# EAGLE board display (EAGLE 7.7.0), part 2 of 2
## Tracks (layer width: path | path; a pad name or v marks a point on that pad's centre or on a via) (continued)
N$131 (continued)
  Top 0.2: 54.6,23.5 1.9,23.5 1.9,23.4 | 1.9,23.4 2.3,23.3 | 2.3,23.3 2.2,23.1 | 2.2,23.1 2.2,23.2 | 2.2,23.2 1.9,23.4 | 2.3,23.3 2.3,23 2.2,22.8 | 1.9,23.4 1.9,20 3.3,20 3.3,22.9 | 2.7,22.1 2.7,22.3 3.3,22.9 | 3.6,23.3 3.7,23.3 3.3,22.9 | 3.6,23.3 3,22.7 2.4,22.7 2.2,22.9 | 2.2,22.9 1.9,23.2 1.9,21.6 | 1.9,21.6 1.9,20.8 2,20.7 2.2,20.7 2.6,20.3 2.6,20.7 | 2.6,22.1 2.6,22.6 3.1,23.1 | 3.1,23.1 3.1,23 | 3.1,23 3.1,22.3 | 3.1,22.3 3,22.2 3,22 2.9,22 2.8,22.1 2.8,23.1 2.9,23.2 | 2.6,21.6 1.9,21.6 | 1.9,21.6 2.3,21.8 2.2,23.2 | 2.2,23.2 2.1,23.2 | 2.1,23.2 1.9,23.4 | 1.9,23.4 54,23.4 | 54,23.4 56.3,23.4 | 56.3,23.4 56.3,26.2 54.4,26.2 54.4,23.5 54.5,23.5 54.6,23.6 | 54.6,25.7 54.6,25.9 54.5,26 56.2,26 56.2,25.6 | 56.2,24.4 56.2,24.2 | 56.2,24.2 56.2,23.5 | 56.2,23.5 54.7,23.5 54.6,23.6 | 54.6,23.6 54.6,23.9 | 54.6,23.9 54.6,24 | 54.6,24.1 54.6,24.4 | 54.6,24.4 54.6,25.7 | 54.6,25.7 54.8,25.9 55.9,25.9 56,25.8 56,24.1 | 56,24.1 56,23.7 54.7,23.7 54.7,23.8 54.6,23.9 | 54.6,23.9 56.1,23.9 56.1,24.1 56.2,24.2 | 56.2,24.2 56.1,24.2 | 56.1,24.2 55.6,24.2 | 55.6,24.2 54.7,24.2 54.6,24.1 | 56,24.1 54.7,24.1 54.6,24 | 54.6,24 54.6,24.1 | 54.6,24.4 54.8,24.4 | 54.8,24.4 56.2,24.4 | 56.2,24.4 56.2,25.6 | 56.2,25.6 56.1,25.7 55.9,25.7 | 55.9,25.7 55.5,25.7 | 55.5,25.7 54.8,25.7 | 54.8,25.7 54.7,25.6 55,25.6 | 55,25.6 55.2,25.6 | 55.2,25.6 55.3,25.6 | 55.3,25.6 55.8,25.6 | 55.8,25.6 55.9,25.7 | 55.9,25.7 56.1,25.9 56.1,25.5 | 56.1,24.2 56.1,25.5 | 56.1,25.5 55.9,25.7 | 55.9,25.7 55.9,25.5 | 55.9,24 55.9,25.5 | 55.9,25.5 55.8,25.6 | 55.8,25.6 55.8,25.4 | 55.8,23.8 55.8,25.4 | 55.8,25.4 55.5,25.7 | 55.5,25.7 55.5,24.3 55.6,24.2 | 55.6,24.2 55.6,25.7 55.5,25.8 55.3,25.6 | 55.3,25.6 55.3,24.4 55.4,24.3 55.4,25.4 55.2,25.6
  Top 0.2: 55.2,25.6 55.2,24.4 55.3,24.3 55.3,25.3 55,25.6 | 55,25.6 55,25.5 | 55,24.3 55,25.5 | 55,25.5 54.8,25.7 | 54.8,25.7 54.8,24.4 | 56.3,23.4 56.3,23.3 | R7A.2 2.4,22.95 2.65,23.2 2.9,23.2 | 2.9,23.2 34.4,23.2 | 34.4,23.2 34.5,23.2 | 34.5,23.2 34.6,23.3 54.3,23.3 | 54.3,23.3 54.4,23.3 | 55.5,23.3 56.3,23.3 | 54.35,23.45 54.4,23.3 | 54.4,23.3 55.5,23.3 | 55.5,23.3 55.5,24.62 JP16.7 54.3,23.42 54.3,23.3 | 2.4,21.9 2.1,23.2 | 2.1,23.2 2.2,23.3 | 2.2,23.3 3.1,23.3 3.1,23.1 | 3.1,20.3 3.1,20.1 2.6,20.7 | 2.6,20.7 2.6,22.1 | 2.6,22.1 2.2,23.3 | 2.9,23.2 2.9,22.8 | 2.9,22.1 2.9,22.8 | 2.9,22.8 2.6,23.1 2.2,23.1 | 2.2,23.1 2,22.9 2,22.1 2.2,22.1 2.2,22.9 | 2.2,22.9 2.6,22.9 2.7,22.8 | 34.2,23.3 34.3,23.3 34.4,23.2 | 34.5,23.2 56.3,23.2 56.3,23.3 | 56.3,23.4 56.2,23.5 | 54.6,24 54,23.4 | 3.6,23.3 3.4,23.3 3.1,23 | 3.1,22.3 3.1,20.3 | 3.1,20.3 2.9,20.1 2.1,20.1 2,20.2
N$134  (1 unrouted)
  Top 0.2: 58.2,26.8 58.4,26.6 | 58.4,26.6 58.6,26.4 | 56.9,26.9 57.1,26.7 | 57.7,26.1 57.1,26.7 | 57.1,26.7 57.3,26.7 57.3,23.2 58.5,23.2 58.6,23.3 | 58.6,23.3 58.7,23.4 58.7,26.5 58.3,26.9 57.5,26.9 57.5,26.8 | 57.5,26.8 57.5,23.4 57.6,23.3 58.3,23.3 | 58.3,23.3 58.6,23.3 | 58.6,23.3 58.6,26.3 58.2,26.7 58.1,26.7 | 58.1,26.7 57.8,26.7 | 57.8,26.7 57.7,26.7 57.7,23.4 57.9,23.4 | 58,23.4 58,23.2 | 58,23.2 58.8,23.2 58.8,26.6 58.4,27 1.1,27 1.1,19.4 | 1.1,19.4 1.1,16.7 3.2,16.7 3.2,18.8 1.4,18.8 1.3,18.9 | R6B.2 1.45,17.8 1.2,18.05 1.2,19 | 1.2,19 1.2,23.55 | 57.65,25.2 57.9,24.95 | 1.3,18.9 1.2,19 | 1.3,18.9 1.3,17 1.1,16.8 | 1.1,16.8 1.1,18 | 1.5,16.8 1.1,16.8 | 58,26.7 58,26.6 | 58,26.6 58,24.82 JP16.6 | 58,23.2 57.4,23.2 57.4,26.8 1.5,26.8 | 1.5,26.8 1.2,26.8 | 1.1,26.9 1.2,26.8 | 1.2,26.8 1.2,26.5 | 1.2,26.5 1.5,26.8 | 1.2,26.5 1.2,18.9 1.4,18.7 | 57.9,23.4 58,23.4 | 58,23.4 58,26.3 57.5,26.8 | 57.5,26.8 57.7,26.8 57.8,26.7 | 57.8,26.7 57.8,23.5 57.9,23.4 | 58,23.4 58.1,23.4 | 58.1,23.4 58.2,23.4 | 58.2,23.4 58.3,23.3 | 58.3,23.3 58.3,26.5 58.2,26.6 58.2,23.5 58.1,23.4 | 58.2,23.4 58.4,23.4 58.4,26.2 | 58.4,26.2 58.5,26.3 | 1.1,19.4 1.8,18.7 1.7,18.7 1.3,19.1 | 58.1,26.7 58,26.6 | 58.4,26.6 58.4,26.2
N$135
  Top 0.2: 2,24.8 2,24.2 | 2,24.2 1.9,24.2 1.9,26.1 53.7,26.1 53.7,24.2 2,24.2
N$137
  Top 0.2: 8.1,19.1 13.1,19.1 | 13.7,19.1 13.1,19.1 | 13.1,19.1 12.8,19.4 12.6,19.4 12.4,19.2
N$138
  Top 0.2: 8.1,18.9 13.7,18.9
N$139
  Top 0.2: 8.1,18.8 13.5,18.8
N$140
  Top 0.2: 8.1,18.4 13.1,18.4 13.3,18.6 8.5,18.6 8.4,18.5 8.4,18.4 8.3,18.3 | 13,18.3 8.3,18.3 | 8.3,18.3 8.1,18.1 12.8,18.1 | 12.8,18.1 12.9,18.2 | 12.8,18.1 12.7,18 8.4,18 8.3,17.9
N$141
  Top 0.2: 13.8,17.7 14.5,17.7 | 15.6,17.7 14.5,17.7 | 14.5,17.7 14.3,17.9
N$142
  Top 0.2: 39.2,19.1 43.4,19.1 44,19.7 | 44,19.7 43.3,19.7 | 43.3,19.7 43.2,19.7 42.7,19.2 42.8,19.2 43.3,19.7 | 44,19.7 44.1,19.7 43.6,19.2 | 43.6,19.2 43,19.2 43.4,19.6 43.6,19.6 | 43.7,19.6 43.6,19.6 | 43.6,19.6 43.3,19.3 43.5,19.3 43.6,19.2 | 43.6,19.2 43.7,19.2 | 43.7,19.2 43.8,19.3 43.8,19.1 38.8,19.1 38.7,19 | 43.7,19.2 43.7,19 43.8,18.9 38.9,18.9 38.8,18.8 38.7,18.8
N$143
  Top 0.2: 24.5,17.7 26,17.7
N$144
  Top 0.2: 62.1,22.4 66.6,22.4 66.8,22.2 62,22.2 62,22.3 61.9,22.3 61.8,22.2
N$145
  Top 0.2: 46.5,17.5 46.1,17.5
N$146
  Top 0.2: 49.9,17.5 54.7,17.5 55.2,18
N$147
  Top 0.2: 66,9 65.7,9 65.6,8.9 65.6,6.6 64.9,5.9 63.5,5.9 63.4,5.8 63.4,4.6 63.1,4.3 60.9,4.3 60.8,4.2 60.8,0.3 73.6,0.3 | 73.7,8.8 73.7,8.5 73.7,0.3 73.6,0.3 | 73.6,0.3 73.6,8.7 73.7,8.8 | 73.7,8.8 65.8,8.8 | 65.7,8.8 65.8,8.8 | 65.8,8.8 66,9 | 66,9 73.6,9 73.7,8.9 73.7,8.8
N$148
  Top 0.2: 60.8,19.3 66.9,19.3 67.7,18.5 60.5,18.5 | 60.5,18.5 60.3,18.7 60.5,18.7 | 59.6,17.4 60.6,17.4 60.8,17.6 67.3,17.6 67.4,17.5 | 67.4,17.5 67.5,17.5 67.6,17.4 67.5,17.4 | 67.5,17.4 67.4,17.5 | 67.5,17.4 67.6,17.3 67.6,16.8 | 67.6,16.8 67.9,16.8 | 69.2,16.8 69.2,17.2 69,17.4 69,18.9 | 69,18.9 68.6,18.9 | 68.6,18.9 67.5,18.9 67,19.4 60.8,19.4 60.3,18.9 | 60.3,18.9 60,18.6 | 67.6,18.7 67.3,18.7 | 67.3,18.7 60.5,18.7 | 60.5,18.7 60.3,18.9 | 60.3,18.9 60.5,18.9 | 60.5,18.9 67.1,18.9 67.3,18.7 | 67.3,18.7 67.3,18.8 67,19.1 60.7,19.1 60.5,18.9 | 60.5,18.9 60.5,19 60.7,19.2 | 60.5,18.5 60.1,18.5 | 67.7,17.3 67.7,16.9 67.6,16.8 | 67.6,16.8 67.6,16.5 69.2,16.5 69.2,16.8 | 69.2,16.8 67.9,16.8 | 67.9,16.8 67.8,16.7 | 67.8,16.7 68.8,16.7 | 68.8,16.7 68.9,16.6 69,16.6 69.1,16.7 68.8,16.7 | 67.8,16.7 67.7,16.6 | 68.6,18.8 68.6,18.9 | 69,18.9 69.1,18.9 69.1,17.2
N$149
  Top 0.2: 60,18.4 67.2,18.4 67.7,17.9 60,17.9 59.9,18 59.9,18.2 60,18.3 67.1,18.3 67.4,18 60.1,18 60,18.1 67.1,18.1
N$150
  Top 0.2: 59.9,17.9 59.9,17.6 | 59.9,17.6 59.8,17.5 | 59.9,17.6 60.7,17.6 60.9,17.8 | 60.9,17.8 67.5,17.8 67.7,17.6 67.4,17.6 67.3,17.7 | 60.9,17.8 60,17.8
N$151
  Top 0.2: 71.1,21.5 71,21.5 70.5,22 70.5,23.2 | 70.5,23.2 70.1,23.6 70.1,26.2 70.5,26.2 | 70.5,26.2 70.7,26.2 | 70.7,26.2 70.8,26.2 | 70.8,26.2 71.8,26.2 71.9,26.1 71.9,20.2 71.9,20.1 | 71.9,20.1 70.5,20.1 | 70.5,20.1 70.5,22.1 70.6,22.2 | 70.8,26.2 70.8,23.3 | 70.8,23.3 70.8,22 | 70.7,26.2 70.7,21.9 | 70.5,26.2 70.5,23.5 | 70.5,23.5 70.5,23.2 | 70.5,23.2 70.6,23.1 | 70.3,26.1 70.3,23.7 70.5,23.5 | 70.8,23.3 70.6,23.3 70.2,23.7 | 70.7,20.5 70.7,20.3 70.5,20.1 | 70.5,20.1 70.6,20 71.9,20 71.9,20.1
N$152
  Top 0.2: 71.7,26.1 71.7,20.7 71.6,20.6
N$153
  Top 0.2: 71.5,26.1 71.5,20.6
N$154
  Top 0.2: 71.4,26.1 71.4,21
N$155
  Top 0.2: 71.2,26.1 71.2,21.8 71.1,21.7
N$156
  Top 0.2: 71,26.1 71,21.8
N$157
  Top 0.2: 63.9,4.8 63.8,4.8 63,4 63.2,4 63.6,4.4
N$158
  Top 0.2: 66.8,20.5 67.6,20.5 67.7,20.4
N$159
  Top 0.2: 67.8,20.7 66.8,20.7
N$160
  Top 0.2: 67.8,20.9 66.3,20.9
N$161
  Top 0.2: 66.8,21.1 67.7,21.1 67.8,21
N$162
  Top 0.2: 67.8,21.3 66.7,21.3
N$163
  Top 0.2: 66.7,21.5 67.7,21.5
N$164
  Top 0.2: 67.9,21.7 66.8,21.7
N$166
  Top 0.2: 65.8,6.5 65,5.7 65.1,5.7 65.6,6.2 65.6,6 65.4,5.8 65.7,5.8 65.8,5.9
N$167
  Top 0.2: 40.2,20.9 39.9,20.9
N$168  (1 unrouted)
  Top 0.2: 4.7,20.5 4.7,20.1 5.6,20.1 5.7,20 | 4.8,21.4 4.8,21.7 4.5,22 4.5,22.4 4.6,22.4 | R7A.1 5.2,21.18 LED6.10 8.2,21.18 8.2,22.5 | 13.3,22.5 13.8,22.5 | 13.8,22.5 16.5,22.5 | 16.5,22.5 16.6,22.5 | 16.7,22.5 18.4,22.5 | 18.4,22.5 18.4,21.2 | 18.4,21.2 17.69,21.2 LED5.10 18.4,21.18 18.4,21.2 | 18.8,22.5 18.9,22.5 | 18.9,22.5 26.7,22.5 | 26.7,22.5 28.6,22.5 | 28.6,22.5 28.6,22.2 | LED4.10 28.6,21.18 28.6,22.2 | 28.6,22.5 28.9,22.5 | 29.1,22.5 36.9,22.5 | 36.9,22.5 38.8,22.5 | 38.8,22.5 38.8,21.2 | 38.8,21.2 38.09,21.2 LED3.10 38.8,21.18 38.8,21.2 | 39.4,22.5 47,22.5 | 47.2,22.5 49,22.5 | 49,22.5 49,21.2 | 49,21.2 48.29,21.2 LED2.10 49,21.18 49,21.2 | 49,22.5 49.3,22.5 | 58.9,22.5 59.2,22.5 | 59.2,22.1 59.2,21.4 | 59.2,21.2 58.49,21.2 LED1.10 | 4.7,22.4 8.1,22.4 8.2,22.5 | 8.2,22.5 4.5,22.5 | 4.5,22.5 4.5,20 5.7,20 | 5.7,20 5.8,20 | 5.8,20 6.2,20.4 12.4,20.4 13.1,21.1 13.1,21.8 13.8,22.5 | 4.7,22.4 4.7,22.2 8.1,22.2 8.1,22 4.8,22 4.7,22.1 4.7,22.3 4.6,22.4 | 8.2,22.5 13.3,22.5 | 13.3,22.5 13.5,22.3 13.4,22.3 13.3,22.4 | 4.7,22.4 4.6,22.4 | 4.6,22.4 4.5,22.5 | 4.5,22.5 4.5,22.6 | 59.2,22.5 60.4,22.5 59.2,21.2 | 59.2,22.5 59.2,22.1 | 59.2,22.1 59.1,22 58.4,22 58,21.6 57.1,22.5 58.9,22.5 | 58.9,22.5 59.1,22.3 57.5,22.3 57.4,22.4 57.4,22.3 57.7,22 59,22 59.1,22.1 57.7,22.1 57.7,22.2 | 48.8,21.8 49.5,22.5 | 49.5,22.5 49.3,22.5 | 49.3,22.5 49.1,22.3 48.3,22.3 47.7,21.7 47.7,21.8 47,22.5 | 47,22.5 47.2,22.5 | 47.2,22.5 47.7,22 48.7,22 48.9,22.2 48.9,22.1 48.8,22 47.9,22 47.5,22.4 48.7,22.4 48.7,22.1 47.9,22.1 47.7,22.3 48.5,22.3 48.6,22.2 | 38.4,21.8 38.7,21.8 39.4,22.5 | 39.4,22.5 38.8,22.5 | 36.9,22.5 37.6,21.8 37.6,21.9 37.5,22 38.7,22 39.1,22.4 37.3,22.4 37.3,22.3 37.4,22.2
  Top 0.2: 37.4,22.2 37.5,22.1 37.4,22.1 37.1,22.4 38.5,22.4 38.7,22.2 37.4,22.2 | 27.6,21.7 27.5,21.7 26.9,22.3 | 26.9,22.3 26.7,22.5 | 28.1,21.6 28.2,21.6 29.1,22.5 | 29.1,22.5 28.9,22.5 | 28.9,22.5 28.7,22.3 27.1,22.3 | 26.9,22.3 27.1,22.3 | 27.1,22.3 27.4,22 28.4,22 28.6,22.2 | 28.6,22.2 27.5,22.2 27.4,22.1 | 17.7,21.7 18,21.7 18.8,22.5 | 18.8,22.5 18.4,22.5 | 16.6,22.5 16.6,22.4 | 16.6,22.4 17.3,21.7 17.3,21.9 16.7,22.5 | 16.7,22.5 16.6,22.5 | 16.5,22.5 16.6,22.4 | 17.9,21.8 18.2,21.8 18.9,22.5 | 59.2,21.2 59.2,21.4 | 59.2,21.4 60.3,22.5 59.4,22.5 59.4,22 | 59.4,21.8 59.3,21.7 59.3,21.8 59.9,22.4 59.6,22.4 59.5,22.3 59.5,22.1 | 59.5,22.1 59.4,22 | 59.4,22 59.7,22 60.1,22.4 60,22.4 59.4,21.8 | 59.4,21.8 59.4,22 | 59.5,22.1 59.7,22.3 | 5.8,20 5.9,20 6.5,20.6 6.3,20.6 5.8,20.1 5.6,20.3 | 4.7,22.4 4.5,22.6 | 4.5,22.6 49.5,22.6 49.5,22.5
N$169
  Top 0.2: 54.9,20.8 54.5,20.8 54.1,20.4 49.8,20.4
N$170
  Top 0.2: 18.2,18.9 18.2,19.2 18.3,19.3 21.6,19.3 22.2,19.9 26.1,19.9 26.7,19.3 | 26.7,19.3 27,19 27,17.9 27.6,17.9 27.7,18 27.7,19.1 27.9,19.3 26.9,19.3 | 26.7,19.3 26.9,19.3 | 26.9,19.3 27.1,19.1
N$171
  Top 0.2: 36.3,21.8 36.3,20.8 36.4,20.7
N$172  (1 unrouted)
  Top 0.2: 18.1,18 18.3,18 18.4,17.9 18.5,17.9 19,18.4 23,18.4 23.5,18.9 | 28.7,18.1 29.2,18.6 29,18.6 28.7,18.3 28.7,18.7 28.6,18.8 33.2,18.8 33.45,19.05 | 28.5,17.9 28.7,17.9 29.3,18.5 33.3,18.5 | 33.3,18.5 33.7,18.9 33.7,19.2 34.3,19.8 | 28.5,19.3 30.5,19.3 31.1,19.9 34.3,19.9 | 43.8,18.7 38.1,18.7 38,18.8 | 38,18.8 38.6,18.8 38.8,18.6 39,18.6 | 43.7,18.6 39,18.6 | 39,18.6 38.8,18.4 43.5,18.4 43.6,18.5 39.3,18.5 38.9,18.1 | 38,18.8 37.4,18.8 37.3,18.9 37.4,18.9 37.8,19.3 36.9,19.3 | 54.3,19.4 54.3,19.5 | 48.8,17.9 49.1,17.9 49.8,18.6 54.3,18.6 54.4,18.7 54.4,19.5 | LED1.9 58.23,18.9 57.8,18.9 57.5,19.2 57.5,17.9 57.7,17.9 | LED2.9 | LED3.9 | R6B.1 5.2,18.5 5,18.5 5,18.64 LED6.9 13.55,18.64 13.8,18.89 13.8,19.9 16,19.9 17.1,18.8 17.53,18.8 LED5.9 | 17.69,18.7 LED5.9 | LED5.9 23.25,18.64 23.5,18.89 23.5,18.9 | LED2.9 54.35,18.64 54.35,19.35 | 54.35,19.35 54.3,19.4 | 54.3,19.4 54.4,19.5 | 48.8,19.3 54.3,19.3 54.35,19.35 | 58.7,19.3 57.6,19.3 | 57.5,19.3 57.6,19.3 | 57.6,19.3 57.7,19.2 57.7,17.9 | 57.7,17.9 58.1,17.9 58.5,18.3 | 54.3,19.4 50.1,19.4 49.6,18.9 49.2,18.9 49,19.1 49.4,19.1 | 49.8,19.1 53.9,19.1 54.3,19.5 | 54.3,19.4 54.3,19 49.5,19 49.4,19.1 | 49.4,19.1 49.8,19.1 | 49.8,19.1 50.2,19.5 54.3,19.5 | 54.3,19.5 54.4,19.5 | LED2.9 47.64,18.64 47.4,18.4 47.4,18.6 47.2,18.8 47.2,19.3 | 47.6,19.3 47.2,19.3 | 47.2,19.3 46.7,19.8 43.8,19.8 43.4,19.4 43.6,19.4 43.7,19.5 43.4,19.5 42.8,18.9 38.35,18.9 LED3.9 | 33.45,19.05 33.45,18.64 LED4.9 27.55,18.74 27.36,18.74 26.9,19.2 26.8,19.2 26.2,19.8 24,19.8 23.5,19.3 23.5,18.9 | 33.45,19.05 33.5,19.1 | 33.5,19.1 34.2,19.8 | 34.2,19.8 34.3,19.8 | 34.3,19.8 36.4,19.8 36.9,19.3
  Top 0.2: 36.9,19.3 37.2,19 37.2,18.6 | 37.2,18.6 37.3,18.5 37.95,18.5 LED3.9 | 37.3,19 37.3,18.7 37.2,18.6 | 37.2,18.6 37.2,18 37.3,17.9 | 34.2,19.8 34.3,19.9 | 34.3,19.9 36.4,19.9 37.2,19.1 | 33.5,19.1 33.5,18.9 33.3,18.7 33.3,19 | 33.4,19.1 34,19.7 31,19.7 30.6,19.3 33.5,19.3 33.7,19.5 31,19.5 30.9,19.4 30.7,19.4 30.5,19.2 33.4,19.2 33.4,19.1 | 33.4,19.1 33.3,19 | 33.3,19 28.7,19 28.7,19.1 31,19.1 | 28.8,18.3 33.1,18.3 33.3,18.5 | 23.5,18.9 23.2,18.9 | 23.1,18.8 22.8,18.5 18.9,18.5 18.5,18.1 18.5,18.4 18.6,18.5 | 18.6,18.5 18.6,18.4 18.4,18.2 18.5,18.2 18.8,18.5 18.6,18.5 | 18.6,18.5 18.3,18.8 23.1,18.8 | 23.1,18.8 23.2,18.9 | 23.2,18.9 23.4,19.1 23.4,19.3 23.9,19.8 22.3,19.8 21.8,19.3 22.1,19.3 | 22.1,19.3 23.2,19.3 23.6,19.7 22.5,19.7 22.4,19.6 | 22.1,19.3 22.2,19.4 | 22.3,19.5 22.4,19.6 | 22.4,19.6 22.4,19.7 | 22.4,19.7 22.3,19.7 | 22.3,19.7 22.1,19.7 21.6,19.2 21.8,19.2 22.3,19.7 | 22.4,19.7 23.2,19.7 23.3,19.6 22.5,19.6 22.4,19.5 | 22.4,19.5 23.2,19.5 | 22.4,19.5 22.3,19.5 | 22.3,19.5 22.2,19.4 | 22.2,19.4 22.2,19 23,19 23.1,19.1 | 23.2,19.2 23.3,19.3 18.7,19.3 18.5,19.1 23.1,19.1 | 23.1,19.1 23.2,19.2 | 23.2,19.2 23.2,18.9 | 23.2,18.9 18.6,18.9 18.5,19
N$173
  Top 0.2: 16.7,19.2 17.3,19.2 17.2,19.3 16.6,19.3 | 16,19.8 16.1,19.8 16.6,19.3 | 16.7,19.2 17.1,18.8 | 16.7,19.2 16.6,19.3
N$174
  Top 0.2: 29.9,21.2 35,21.2 35.3,21.5 35.3,21.9 | 26.1,21.8 26.1,20.5 | 26.1,20.5 25.6,20.5 | 25.6,20.5 24.9,20.5 | 24.9,20.5 24.8,20.6 25.5,20.6 25.6,20.5 | 24.7,21.8 24.8,21.8 24.9,21.9 | 24.9,21.9 25.8,21.9 | 25.8,21.9 26.2,21.9 26.3,21.8 26.3,20.5 | 35,21.8 35,21.9 | 35,21.9 35.3,21.9 | 35.3,21.9 36.4,21.9 36.5,21.8 36.5,20.5 | 34.8,20.7 34.8,20.5 | 45.3,20.7 39.8,20.7 39.8,20.8 | 45.8,20.5 46.7,20.5 | 45.7,21 45.7,20.6 45.8,20.5 | 68,21.3 68.4,21.3 69.1,22 69.1,22.1 65.9,22.1 | 65.9,22.1 65.3,22.1 | 65.3,22.1 65.3,21.7 | 65.3,21.7 65.3,21.2 | 65.3,21.1 65.3,20.8 | 65.3,20.8 65.3,20.6 | 65.3,20.6 65.3,20.3 65.5,20.3 | 65.5,20.3 69.1,20.3 69.1,20.1 | 69.1,20.1 65.7,20.1 | 65.2,20.2 65.6,20.2 65.7,20.1 | LED6.1 15.11,21.09 15.7,20.5 16.2,20.5 | LED1.1 68.4,21.18 R1G.1 | 25.33,21.2 LED5.1 | 35.49,21.2 LED4.1 | 45.69,21.2 LED3.1 39.85,21.18 39.85,20.85 39.8,20.8 | 55.89,21.2 LED2.1 | 66.09,21.2 LED1.1 | 19.2,20.93 19.25,21.18 LED5.1 | LED4.1 29.85,21.18 29.85,20.35 | 49.6,20.93 49.85,21.18 LED2.1 | 16.2,20.5 16.8,19.9 18.9,19.9 | 19.2,20.4 19.2,20.2 18.9,19.9 | 19.2,20.4 19.2,20.5 | 19.2,20.5 19.2,20.7 | 19.2,20.8 19.2,20.93 | 15.4,21.2 15.5,21.2 16.2,20.5 | LED1.1 60.68,21.18 | 60.68,21.18 60.4,20.9 | 60.4,20.9 59.6,20.1 | 59.5,20 57.5,20 | 57.5,20 57,20.5 | 57,20.5 56.7,20.8 56.29,20.8 LED2.1 | 65.7,20.1 59.6,20.1 | 59.6,20.1 59.5,20 | 59.5,20 69.1,20 69.1,20.1 | 60.68,21.18 61.4,21.9 | 61.4,21.9 65.7,21.9 65.9,22.1 | 65.3,22.1 61.6,22.1 | 61.6,22.1 61.4,21.9 | 59.9,20.2 60.2,20.2 | 60.2,20.2 65.4,20.2 65.5,20.3 | 65.5,20.3 65.4,20.4 60.1,20.4 | 60,20.4 60.1,20.4 | 60.1,20.4 60.2,20.5 65.2,20.5 65.3,20.6 | 60.3,20.7 65.2,20.7 65.3,20.8 | 65.3,20.8 60.5,20.8 60.4,20.9
  Top 0.2: 60.4,20.9 65.1,20.9 65.3,21.1 | 65.3,21.1 65.4,21.2 | 65.4,21.2 65.3,21.2 | 61.1,21.2 60.8,21.2 60.7,21.1 65.3,21.1 | 65.3,21.1 65.3,21.2 | 65.3,21.2 61.1,21.2 | 61.1,21.2 61,21.3 65.3,21.3 65.4,21.2 | 65.4,21.2 65.4,21.4 61.1,21.4 61.1,21.5 61.2,21.6 65.5,21.6 65.6,21.5 65.5,21.5 65.3,21.7 | 65.3,21.7 61.7,21.7 | 61.7,21.7 61.4,21.7 | 55.3,20.5 56.9,20.5 | 57,20.5 56.9,20.5 | 56.9,20.5 56.7,20.7 56.7,21.9 50.3,21.9 49.7,21.3 | 49.6,21 49.7,20.9 49.7,21.1 50.4,21.8 55.2,21.8 55.3,21.7 55.3,21.3 | 55.3,21 55.3,20.5 | 55.3,20.5 50,20.5 50,20.7 55.1,20.7 55.1,20.8 55.2,20.9 50.3,20.9 | 50.3,20.9 49.9,20.9 | 49.9,20.9 49.9,21 50,21.1 50.1,21.1 | 50.1,21.1 55.2,21.1 55.3,21 | 55.3,21 55.3,21.3 | 55.3,21.3 55.2,21.4 50.3,21.4 50.2,21.3 50.2,21.4 50.4,21.6 55.3,21.6 55.4,21.5 55.4,21.3 49.7,21.3 | 57.5,20 57.6,19.9 59.4,19.9 | 59.4,19.9 59.5,20 | 59.4,19.9 59.9,19.9 60.2,20.2 | 49.7,21.3 49.6,21.2 49.6,20.2 | 49.6,20.2 49.3,19.9 47.3,19.9 46.7,20.5 | 46.7,20.5 46.1,21.1 | 50.3,20.9 49.6,20.2 | 50.1,21.1 50.1,20.9 49.7,20.5 49.7,20.8 49.8,20.8 49.9,20.9 | 46.7,20.5 46.7,21.6 | 46.7,21.6 46.4,21.9 46.4,20.9 46.6,20.7 46.6,21.6 46.7,21.6 | 46.7,21.6 46.7,21.7 46.5,21.9 46.5,21.6 45.3,21.6 45,21.9 40.4,21.9 39.7,21.2 39.7,20.7 | 39.7,20.7 39.7,20.3 39.5,20.1 | 39.5,20.1 39.3,19.9 | 39.3,19.9 37.1,19.9 36.5,20.5 | 36.4,20.5 35.72,21.18 LED4.1 | 39.8,20.8 39.7,20.7 | 39.3,19.9 41.6,19.9 42.2,20.5 45.8,20.5 | 45.8,20.5 45.9,20.6 | 39.8,20.8 45,20.8 45.1,20.9 45.1,21 40,21 40,21.3 45.3,21.3 45.2,21.4 40.1,21.4 | 40,21.4 40.1,21.4 | 40.1,21.4 40.2,21.5 40.3,21.5 | 40.3,21.5 45.3,21.5 | 45.5,21.5 45.3,21.5 | 45.3,21.5 45.1,21.7 40.5,21.7
  Top 0.2: 40.3,21.5 40.5,21.7 | 40.5,21.7 40.3,21.7 40.2,21.6 | 39.5,20.1 41.6,20.1 42.1,20.6 40,20.6 39.9,20.5 39.8,20.6 39.8,20.2 41.6,20.2 41.9,20.5 40.1,20.5 39.9,20.3 41.6,20.3 41.7,20.4 | 34.8,20.5 35.9,20.5 | 35.9,20.5 36.4,20.5 | 36.4,20.5 36.5,20.5 | 29.7,20.2 29.4,19.9 29.2,19.9 | 29.1,19.9 26.9,19.9 26.3,20.5 | 26.3,20.5 25.9,20.9 25.59,20.9 LED5.1 | 26.1,20.5 26.3,20.5 | 35,21.9 30.1,21.9 29.7,21.5 29.7,20.5 29.1,19.9 | 29.1,19.9 29.2,19.9 | 29.2,19.9 29.5,20.2 29.7,20.2 | 29.7,20.2 29.85,20.35 | 29.85,20.35 30.2,20.7 35.7,20.7 35.9,20.9 35.9,20.5 | 34.8,20.5 29.9,20.5 29.8,20.4 29.8,20.6 30,20.8 30.2,20.8 | 30.2,20.8 35.1,20.8 35.2,20.9 30,20.9 29.9,21 34.9,21 35,21.1 35,21.4 29.9,21.4 | 29.8,21.4 29.9,21.4 | 29.9,21.4 30,21.5 34.8,21.5 34.8,21.6 30.1,21.6 30.2,21.7 | 30.2,21.7 35.1,21.7 | 30.2,21.7 30.1,21.7 29.9,21.5 | 29.9,21.4 29.8,21.3 29.8,21.2 30.2,20.8 | 30.2,20.8 30,20.6 29.9,20.6 29.6,20.3 | 25.8,21.7 25.8,21.9 | 24.9,21.9 19.7,21.9 19.2,21.4 19.2,20.93 | 18.9,19.9 21.1,19.9 21.7,20.5 | 21.8,20.6 21.7,20.5 | 21.7,20.5 24.9,20.5 | 25.2,20.7 19.2,20.7 | 19.2,20.7 19.2,20.8 | 19.2,20.8 24.7,20.8 24.8,20.9 24.8,21 19.4,21 19.3,20.9 19.3,21.3 24.6,21.3 24.8,21.5 19.5,21.5 | 19.5,21.5 19.4,21.4 | 19.5,21.5 19.7,21.7 24.9,21.7 | 19.2,20.5 21.6,20.5 | 19.2,20.4 21.4,20.4 21.4,20.3 21.3,20.2 19.3,20.2 19.2,20.1 19.3,20.1 | 19.3,20.1 21.1,20.1 | 19.3,20.1 19.2,20 | 61.7,21.7 61.7,22 61.6,22.1 | 61.6,22.1 62.1,22.6 66.6,22.6 67.3,21.9 | 66.7,21.9 67.3,21.9 | 67.3,21.9 67.8,21.9
N$175
  Top 0.2: 25.5,18.9 25.9,18.9 26,19 26,18.8 26.1,18.7 26.1,17.7 26.2,17.6 | 36,18.5 36,18.1 36.7,17.4 | 15.3,18.6 15.8,18.6 16.1,18.3 16.1,18.2 | 15.2,19.3 14.4,19.3 14.4,18.4 13.9,17.9 | 13.9,17.9 13.5,17.5 | 57,17.4 59.55,17.4 59.8,17.65 59.8,18.39 60.05,18.64 LED1.2 66.11,18.55 66.36,18.3 67.6,18.3 67.6,18.05 67.85,17.8 R2F.1 | 57,17.4 56.9,17.4 | 56.9,17.4 55.9,17.4 | 55.9,17.4 LED2.2 55.91,17.41 55.9,17.4 | 54.9,17.4 49.6,17.4 | 49.6,17.4 46.9,17.4 | 46.9,17.4 45.8,17.4 | 45.8,17.4 45.7,17.4 | 45.7,17.4 LED3.2 45.71,17.49 45.8,17.4 | 45.7,17.4 39.6,17.4 | 39.6,17.4 36.7,17.4 | 36.5,17.4 35.5,17.4 | 35.5,17.4 LED4.2 35.51,17.41 35.5,17.4 | 35.5,17.4 29.3,17.4 | 29.3,17.4 26.4,17.4 | 26.4,17.4 25.4,17.4 | 25.1,17.4 25.1,18.43 LED5.2 25.31,17.49 25.4,17.4 | 25.4,17.4 25.1,17.4 | 25.1,17.4 19,17.4 | 19,17.4 16.3,17.4 | 16.3,17.4 16.2,17.4 | 15.5,17.4 15.1,17.4 | 15.1,17.4 LED6.2 | 13.5,17.5 15,17.5 15.1,17.4 | 15.1,17.4 13.4,17.4 13.5,17.5 | 13.9,17.9 14,17.9 | 14.1,17.9 14.2,17.9 14.4,18.1 | 15.4,18.4 15.4,18.2 16.2,17.4 | 16.2,17.4 15.5,17.4 | 15.5,17.4 15.3,17.6 15.9,17.6 | 15.9,17.6 15.7,17.8 15.5,17.8 15.2,17.5 | 16.3,17.4 16.1,17.6 16.1,18.2 | 16.1,18.2 15.9,18.4 15.9,17.6 | 15.9,17.6 16,17.5 | 14.7,18.4 14.5,18.4 14,17.9 | 14,17.9 14.1,17.9 | 14.1,17.9 14.2,17.8 13.9,17.8 13.7,17.6 | 19,17.4 19.2,17.6 | 19.2,17.6 19.3,17.7 24.1,17.7 24.6,18.2 | 19.2,17.6 24.2,17.6 | 24.2,17.6 24.5,17.9 | 25.8,18.4 25.8,18 26.2,17.6 | 26.2,17.6 26.3,17.5 26.4,17.4 | 26.2,17.6 24.2,17.6 | 29.3,17.4 29.6,17.7 34.1,17.7 | 34.1,17.7 34.2,17.7 34.8,18.3 34.8,18.1 34.3,17.6 33.9,17.6 | 33.6,17.6 29.6,17.6 29.5,17.5 36.2,17.5 36.3,17.6 36.3,17.7 36.2,17.8 34.7,17.8 34.6,17.7
  Top 0.2: 36.2,17.7 34.6,17.7 | 34.6,17.7 34.5,17.6 | 36.7,17.4 36.5,17.4 | 36.5,17.4 36.4,17.5 | 39.6,17.4 39.8,17.6 44.3,17.6 | 44.3,17.6 45,18.3 46,18.3 46.4,17.9 46.4,17.7 | 46.4,17.7 46.4,17.6 44.5,17.6 | 44.3,17.6 44.5,17.6 | 44.5,17.6 45,18.1 45,17.9 44.9,17.8 46.2,17.8 46.3,17.7 44.7,17.7 | 46.1,18.3 46.1,18.2 46.9,17.4 | 46.4,17.7 46.6,17.5 | 49.6,17.4 49.9,17.7 54.7,17.7 55.3,18.3 | 56.4,18.4 56.4,17.9 56.6,17.7 | 56.6,17.7 56.9,17.4 | 55.9,17.4 54.9,17.4 | 54.9,17.4 54.8,17.5 55.1,17.5 | 56.6,17.5 55.1,17.5 | 55.1,17.5 55,17.6 56.5,17.6 56.6,17.7 | 56.6,17.7 55.1,17.7 | 56.3,18.1 57,17.4 | 34.1,17.7 34.9,18.5 | 33.6,17.6 33.9,17.6 | 33.9,17.6 35,18.7 | 33.6,17.6 34.8,18.8 34.8,18.7 33.9,17.8
N$177
  Top 0.2: 71.7,12 72.8,12 | 72.8,12 73.5,12 | 73.5,12 73.5,11.3 | 73.5,11.3 73.5,10.9 | 73.5,10.7 73.5,10.4 | 63.2,24.4 63.2,23.2 | 63.2,23.2 62.4,23.2 62.4,27.7 73.7,27.7 73.7,10.4 | 73.7,10.4 73.7,10.2 | 73.7,10.2 70.5,10.2 70.5,9.9 73.7,9.9 73.7,10 | 73.7,10 73.7,10.1 | 73.7,10.1 70.7,10.1 70.6,10 70.6,11.8 70.5,11.9 70.5,12.2 73.4,12.2 73.5,12.3 73.5,27.6 | 73.5,10.4 73.7,10.4 | 73.7,10.2 73.7,10.1 | 73.7,10 72.3,10 71.9,10.4 73.5,10.4 | 72.85,11.1 71.9,11.1 | 71.9,11.1 R4D.2 | JP16.4 63.2,25.35 63.1,25.45 63.35,25.7 63.35,26.95 63.6,27.2 63.6,27.3 63.8,27.5 64.4,27.5 | 64.6,27.5 73.2,27.5 | 73.5,27.5 73.2,27.5 | 73.2,27.5 73.6,27.1 73.6,12.8 | 73.6,12.6 73.6,12.2 | 73.6,12.2 73.6,11.85 72.85,11.1 | 73.5,12 73.5,12.1 73.6,12.2 | 73.6,12.2 72.4,12.2 72.1,11.9 72.1,11.3 | 72.1,11.2 72.1,10.5 73.4,10.5 73.4,11.6 | 73.4,11.6 73.4,11.8 72.2,11.8 72.2,11 71.9,10.7 73.5,10.7 | 73.5,10.7 73.5,10.9 | 73.5,10.9 71.8,10.9 71.8,11 71.9,11.1 | 72.85,11.1 73.6,11.1 73.6,11.2 73.5,11.3 | 73.5,11.3 72.2,11.3 72.1,11.2 | 72.1,11.2 72.1,11.3 | 72.1,11.3 71.9,11.5 73.5,11.5 | 73.6,11.5 73.5,11.5 | 73.5,11.5 73.4,11.6 | 73.4,11.6 71.9,11.6 | 72.8,12 73.6,12.8 | 73.6,12.8 73.6,12.6 | 73.6,12.6 73.3,12.3 | 63.2,23.2 63.9,23.2 63.9,26.8 64.6,27.5 | 64.6,27.5 64.4,27.5 | 64.4,27.5 63.6,26.7 63.5,26.7 63.4,26.8 63.5,26.8 63.6,26.9 | 63.6,26.9 64.1,27.4 63.9,27.4 63.4,26.9 63.4,27.3 63.7,27.6 63.1,27.6 | 63.1,27.6 62.6,27.6 62.6,23.4 | 63.8,23.4 63.5,23.4 | 63.5,23.4 62.6,23.4 | 62.6,23.4 62.5,23.3 62.6,23.3 62.8,23.5 62.8,27.5 63,27.5 63.1,27.6 | 63.1,27.6 63.1,27.5 | 63.1,23.8 63.1,23.6 63,23.5 63,27.4 63.1,27.5 | 63.1,27.5 63.1,23.8 | 63.1,23.8 63.3,23.6
  Top 0.2: 63.3,23.6 63.5,23.4 | 63.5,23.4 63.5,27.3 63.3,27.5 63.3,23.6 | 63.3,23.6 63.6,23.6 63.7,23.5 63.7,26.8 63.6,26.9
(copper drawn outside any net)
  shapes: Top area x83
